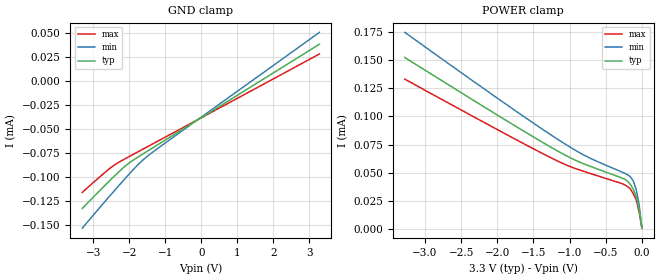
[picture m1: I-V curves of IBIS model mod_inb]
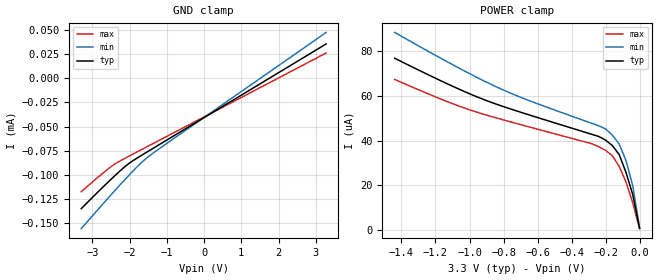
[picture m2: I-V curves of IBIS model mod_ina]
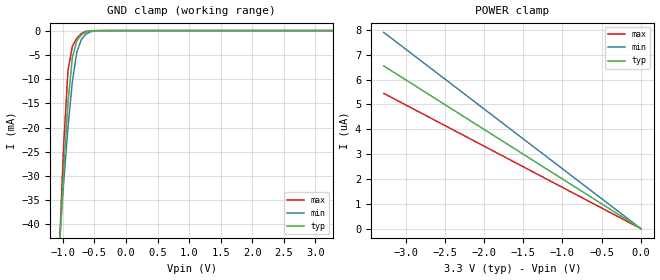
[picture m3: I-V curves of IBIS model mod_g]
| IBIS (I/O, Buffer, Information, Specification) Model, officially
| electronic behavioral standard for Buffer structures of digital pins.
[IBIS ver]  4.2
[File name] rhflvds42_3v3_rev1.ibs
[File Rev]  1.0
[Date]   17 March 2026
[Source]   CAD & Design Services (Catania) - STMicroelectronics
[Notes]
  (Note1) This IBIS model is the model of the product with package
   (Flat16 package elements);
  (Note2) This IBIS model is extracted with nominal 3.3V power supply
   (min:3.00V, typ:3.30V, max:3.60V);
  (Note3) This model has few Notes about the non-monotonicity
   of I-V curves, but they are not indicative of problems
   inside the model;
[Disclaimer]
   Customers are solely responsible for all aspects of their
   own product designs or applications using this IBIS Model.
   STMicroelectronics assumes no liability for Custmer Designs
   and applications associated to this IBIS Model.
   In the use of this IBIS Model Customer shall not modify,
   disassemble, alter this Model in whole or in part.
   If Customers do not accept these terms, the IBIS Model
   may not be used. For any problems or modifications please
   contact STMicroelectronics (www.st.com).
[Copyright] (c) 2026 STMicroelectronics
|   Component RHFLVDS42
[Component] RHFLVDS42
[Manufacturer] STMicroelectronics
[Package]
| variable   typ   min   max
R_pkg   0.0   0.0   0.0
L_pkg   0.0H   0.0H   0.0H
C_pkg   0.0F   0.0F   0.0F
[Pin]  signal_name   model_name   R_pin   L_pin   C_pin
1   1B   mod_inb   0.0   0.0   0.0
2   1A   mod_ina   0.0   0.0   0.0
3   2A   mod_ina   0.0   0.0   0.0
4   2B   mod_inb   0.0   0.0   0.0
5   3B   mod_inb   0.0   0.0   0.0
6   3A   mod_ina   0.0   0.0   0.0
7   4A   mod_ina   0.0   0.0   0.0
8   4B   mod_inb   0.0   0.0   0.0
9   GN   mod_g   0.0   0.0   0.0
10   4Y   mod_y   0.0   0.0   0.0
11   3Y   mod_y   0.0   0.0   0.0
12   GND   GND   0.0   0.0   0.0
13   VCC   POWER   0.0   0.0   0.0
14   2Y   mod_y   0.0   0.0   0.0
15   1Y   mod_y   0.0   0.0   0.0
16   G   mod_g   0.0   0.0   0.0
[Diff pin]  inv_pin   vdiff   tdelay_typ   tdelay_min   tdelay_max
|nA   nB   mV   -   -   -
2   1   100mV   0.0s   0.0s   0.0s
3   4   100mV   0.0s   0.0s   0.0s
6   5   100mV   0.0s   0.0s   0.0s
7   8   100mV   0.0s   0.0s   0.0s
[Package Model]  FE0032_RH_LVDS42
[Define Package Model]  FE0032_RH_LVDS42
[Manufacturer]  STMicroelectronics
[OEM]  STMicroelectronics
[Description]  flat-16
[Number Of Pins]  16
[Pin Numbers]
|Pin Num   Terminal Name
1   | NET1_B1:bw3
2   | NET2_A1:bw4
3   | NET3_A2:bw6
4   | NET4_B2:bw7
5   | NET5_B3:bw9
6   | NET6_A3:bw10
7   | NET7_A4:bw12
8   | NET8_B4:bw13
9   | NET9_GB:bw19
10   | NET10_Y4:bw23
11   | NET11_Y3:bw26
12   | NET12_GND:bw_gnd
13   | NET13_VCC:bw_vcc
14   | NET14_Y2:bw30
15   | NET15_Y1:bw33
16   | NET16_G:bw37
[Model Data]
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[End Model Data]
[End Package Model]
| Models and submodels in the file (4): mod_inb (Input), mod_ina (Input), mod_g (Input), mod_y (3-state)
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|   Model mod_inb
[Model]   mod_inb
Model_type Input
Vinl   =   1.000V
Vinh   =   2.300V
C_comp   11.121pF   10.620pF   11.645pF
[Temperature Range]  25.0000   0.1250k   -55.0000
[Voltage Range]   3.3000V   3.0000V   3.6000V
[GND_clamp]
|Voltage   I(typ)   I(min)   I(max)
-3.3V     -132.4uA   -152.9uA   -115.7uA
-2.46V    -100.6uA   -116.1uA   -88.6uA
-2.04V    -86.27uA   -98.34uA   -79.29uA
-1.55V    -74.16uA   -79.84uA   -69.38uA
3.28V     38.35uA    50.68uA    28.21uA
[POWER_clamp]
|Voltage   I(typ)   I(min)   I(max)
-3.28V    152.4uA    174.7uA    133.1uA
-1.92V    98.08uA    112.6uA    85.55uA
-1.12V    67.63uA    77.81uA    58.95uA
-920mV    61.08uA    69.88uA    53.69uA
-760mV    56.77uA    64.26uA    50.24uA
-240mV    44.23uA    49.6uA     39.29uA
-200mV    42.5uA     48.21uA    37.77uA
-160mV    39.56uA    46.43uA    35.46uA
-120mV    35.42uA    42.75uA    31.45uA
-80mV     29.19uA    35.27uA    26.13uA
-40mV     17.95uA    22.2uA     15.52uA
0V        847nA      928nA      708nA
|   Model mod_ina
[Model]   mod_ina
Model_type Input
Vinl   =   1.000V
Vinh   =   2.300V
C_comp   11.121pF   10.620pF   11.645pF
[Temperature Range]  25.0000   0.1250k   -55.0000
[Voltage Range]   3.3000V   3.0000V   3.6000V
[GND_clamp]
|Voltage   I(typ)   I(min)   I(max)
-3.3V     -135.1uA   -155.9uA   -117.5uA
-2.46V    -103.2uA   -119.1uA   -90.47uA
-2.04V    -88.89uA   -101.4uA   -81.16uA
-1.55V    -76.78uA   -82.85uA   -71.25uA
3.28V     35.72uA    47.66uA    26.34uA
[POWER_clamp]
|Voltage   I(typ)   I(min)   I(max)
|  -3.28   0.1497mA   0.1717mA   0.1312mA
|  -3.24   0.1481mA   0.1699mA   0.1298mA
|  -3.20   0.1465mA   0.1680mA   0.1284mA
|  -3.16   0.1449mA   0.1662mA   0.1270mA
|  -3.12   0.1433mA   0.1643mA   0.1256mA
|  -3.08   0.1417mA   0.1625mA   0.1242mA
|  -3.04   0.1401mA   0.1606mA   0.1228mA
|  -3.00   0.1385mA   0.1588mA   0.1214mA
|  -2.96   0.1369mA   0.1570mA   0.1200mA
|  -2.92   0.1353mA   0.1551mA   0.1186mA
|  -2.88   0.1337mA   0.1533mA   0.1172mA
|  -2.84   0.1321mA   0.1515mA   0.1158mA
|  -2.80   0.1304mA   0.1496mA   0.1144mA
|  -2.76   0.1288mA   0.1478mA   0.1129mA
|  -2.72   0.1272mA   0.1460mA   0.1115mA
|  -2.68   0.1256mA   0.1441mA   0.1101mA
|  -2.64   0.1240mA   0.1423mA   0.1087mA
|  -2.60   0.1224mA   0.1405mA   0.1073mA
|  -2.56   0.1208mA   0.1386mA   0.1059mA
|  -2.52   0.1192mA   0.1368mA   0.1045mA
|  -2.48   0.1176mA   0.1350mA   0.1031mA
|  -2.44   0.1161mA   0.1332mA   0.1017mA
|  -2.40   0.1145mA   0.1313mA   0.1003mA
|  -2.36   0.1129mA   0.1295mA   98.9580uA
|  -2.32   0.1113mA   0.1277mA   97.5630uA
|  -2.28   0.1097mA   0.1259mA   96.1690uA
|  -2.24   0.1081mA   0.1241mA   94.7750uA
|  -2.20   0.1065mA   0.1223mA   93.3830uA
|  -2.16   0.1049mA   0.1204mA   91.9930uA
|  -2.12   0.1033mA   0.1186mA   90.6030uA
|  -2.08   0.1018mA   0.1168mA   89.2150uA
|  -2.04   0.1002mA   0.1150mA   87.8280uA
|  -2.00   98.6010uA   0.1132mA   86.4430uA
|  -1.96   97.0250uA   0.1114mA   85.0590uA
|  -1.92   95.4500uA   0.1096mA   83.6780uA
|  -1.88   93.8790uA   0.1078mA   82.2980uA
|  -1.84   92.3100uA   0.1060mA   80.9200uA
|  -1.80   90.7430uA   0.1043mA   79.5450uA
|  -1.76   89.1800uA   0.1025mA   78.1730uA
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-1.44V    76.83uA    88.39uA    67.33uA
-1.08V    63.61uA    73.16uA    55.91uA
-840mV    56.2uA     63.95uA    50.05uA
-640mV    51.23uA    57.59uA    45.89uA
-280mV    42.74uA    47.66uA    38.53uA
-240mV    41.81uA    46.58uA    37.22uA
-200mV    40.17uA    45.2uA     35.6uA
-160mV    37.73uA    42.42uA    33.19uA
-120mV    33.7uA     38.44uA    28.38uA
-80mV     25.76uA    31.06uA    21.46uA
-40mV     15.73uA    19.68uA    12.05uA
0V        691nA      963nA      538nA
|   Model mod_g
[Model]   mod_g
Model_type Input
Vinl   =   1.000V
Vinh   =   2.300V
C_comp   11.121pF   10.620pF   11.645pF
[Temperature Range]  25.0000   0.1250k   -55.0000
[Voltage Range]   3.3000V   3.0000V   3.6000V
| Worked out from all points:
|   GND clamp passes 1 mA (typ) near -0.72 V on its own axis
[GND_clamp]
|Voltage   I(typ)   I(min)   I(max)
-3.3V     -689mA     -525.7mA   -920.4mA
-1.06V    -46.53mA   -44.55mA   -46.47mA
-990mV    -29.57mA   -31.72mA   -24.16mA
-920mV    -14.98mA   -20.05mA   -8.271mA
-850mV    -5.513mA   -10.5mA    -3.209mA
-780mV    -2.112mA   -4.491mA   -1.575mA
-710mV    -895.4uA   -1.88mA    -630.2uA
-640mV    -328.7uA   -783.6uA   -171.8uA
-570mV    -98.54uA   -280.7uA   -35.77uA
-360mV    -7.802uA   -13.62uA   -6.592uA
3.28V     -39.92nA   675.4nA    -531.3nA
[POWER_clamp]
|Voltage   I(typ)   I(min)   I(max)
-3.28V    6.552uA    7.901uA    5.447uA
-2.72V    5.433uA    6.552uA    4.517uA
-1.88V    3.755uA    4.528uA    3.122uA
0V        31.67pA    1.173nA    28.81pA
